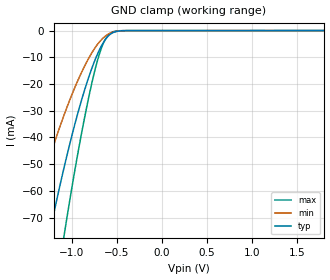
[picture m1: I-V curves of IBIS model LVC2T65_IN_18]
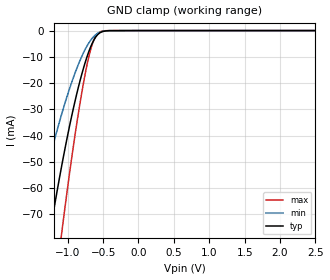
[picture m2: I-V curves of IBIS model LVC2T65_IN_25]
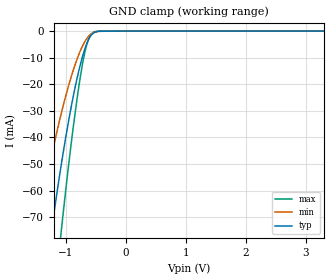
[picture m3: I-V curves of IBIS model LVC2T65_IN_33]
| TEXAS INSTRUMENTS INCORPORATED
| 2-BIT BIDIRECTIONAL VOLTAGE LEVEL TRANSLATOR FOR OPEN DRAIN APPLICATIONS
| Marketing part#   Voltage Range   Package-type   #pins/pkg drawing
| TXS0102DCU   1.65V - 5.5V   TSSOP   8 / DCU
| TXS0102DCT   1.65V - 5.5V   TSSOP   8 / DCT
| TXS0102DQE   1.65V - 5.5V   X2SON   8 / DQE
[IBIS Ver]   3.2
[File Name]   txs0102.ibs
[File Rev]   1.2
[Date]   May 11, 2015
[Source]   Model built from spectre simulations at:
   Texas Instruments Incorporated.
   Webench Design Center
   12500 TI Blvd
   Dallas, TX -75243
   For Support e-mail: elab_ibis@list.ti.com
[Notes]   Revision_History:
   Rev 1.2: Added DGE package component. 5/11/15
   Rev 1.1: Updated Vih/Vih for all buffers. 8/22/12
   Power Clamps and Pullups for IO_A and IO_B are non-monotonic
[Disclaimer] This model is designed as an aid for customers of Texas Instruments
 TI and its licensors and suppliers make no warranties, either expressed
 or implied, with respect to this  model, including the warranties of
 merchantability or fitness for a particular purpose.
 The model is provided solely on an "as is" basis. The entire risk as to
 its quality and performance is with the customer.
[Copyright] (C)Copyright 2015 Texas Instruments Incorporated.
   All rights reserved.
| Component TXS0102_DCU 8-PIN TSSOP
[Component]   TXS0102_DCU
[Manufacturer]   Texas Instruments, Inc.
[Package]
|   typ   min   max
R_pkg   1.400e-02   1.300e-02   1.500e-02
L_pkg   1.289e-09   1.025e-09   2.014e-09
C_pkg   1.360e-13   6.600e-14   2.940e-13
[Pin]   signal_name   model_name   R_pin   L_pin   C_pin
1   B2   LVC2T65_IO_B   1.400e-02   1.387e-09   1.760e-13
2   GND   GND   1.300e-02   1.026e-09   6.600e-14
3   VCCA   POWER   1.300e-02   1.032e-09   6.700e-14
4   A2   LVC2T65_IO_A   1.500e-02   2.014e-09   2.940e-13
5   A1   LVC2T65_IO_A   1.400e-02   1.412e-09   1.780e-13
6   OE   LVC2T65_IN   1.300e-02   1.030e-09   6.600e-14
7   VCCB   POWER   1.300e-02   1.025e-09   6.600e-14
8   B1   LVC2T65_IO_B   1.400e-02   1.386e-09   1.760e-13
| Component TXS0102_DCT 8-PIN TSSOP
[Component]   TXS0102_DCT
[Manufacturer]   Texas Instruments, Inc.
[Package]
|   typ   min   max
R_pkg   2.900e-02   2.800e-02   3.100e-02
L_pkg   1.796e-09   1.666e-09   1.924e-09
C_pkg   1.090e-13   8.300e-14   1.360e-13
[Pin]   signal_name   model_name   R_pin   L_pin   C_pin
1   B2   LVC2T65_IO_B   3.100e-02   1.894e-09   1.340e-13
2   GND   GND   2.800e-02   1.697e-09   8.600e-14
3   VCCA   POWER   3.000e-02   1.722e-09   8.600e-14
4   A2   LVC2T65_IO_A   3.000e-02   1.861e-09   1.300e-13
5   A1   LVC2T65_IO_A   2.800e-02   1.924e-09   1.360e-13
6   OE   LVC2T65_IN   2.900e-02   1.736e-09   8.600e-14
7   VCCB   POWER   2.800e-02   1.666e-09   8.300e-14
8   B1   LVC2T65_IO_B   3.000e-02   1.871e-09   1.320e-13
| Component TXS0102_DQE 8-PIN X2SON
[Component]   TXS0102_DQE
[Manufacturer]   Texas Instruments, Inc.
[Package]
|   typ   min   max
R_pkg   0.0401   0.0391   0.0417
L_pkg   0.3040n   0.2971n   0.3158n
C_pkg   0.0474p   0.0450p   0.0526p
[Pin]   signal_name   model_name   R_pin   L_pin   C_pin
1   VCCA   POWER   0.04056   0.31110n   0.04603p
2   A1   LVC2T65_IO_A   0.03969   0.30316n   0.04651p
3   A2   LVC2T65_IO_A   0.03995   0.30556n   0.05161p
4   GND   GND   0.03907   0.29711n   0.04499p
5   OE   LVC2T65_IN   0.03987   0.29814n   0.04522p
6   B2   LVC2T65_IO_B   0.03990   0.29821n   0.04651p
7   B1   LVC2T65_IO_B   0.04172   0.31579n   0.05261p
8   VCCB   POWER   0.04034   0.30276n   0.04549p
| Model LVC2T65_IN
[Model Selector]   LVC2T65_IN
LVC2T65_IN_18   1.8 volt Vcc
LVC2T65_IN_25   2.5 volt Vcc
LVC2T65_IN_33   3.3 volt Vcc
LVC2T65_IN_50   5 volt Vcc
| Model LVC2T65_IO_A
[Model Selector]   LVC2T65_IO_A
LVC2T65_IO_A_18   1.8 volt Vcc
LVC2T65_IO_A_25   2.5 volt Vcc
LVC2T65_IO_A_33   3.3 volt Vcc
LVC2T65_IO_A_50   5 volt Vcc
| Model LVC2T65_IO_B
[Model Selector]   LVC2T65_IO_B
LVC2T65_IO_B_18   1.8 volt Vcc
LVC2T65_IO_B_25   2.5 volt Vcc
LVC2T65_IO_B_33   3.3 volt Vcc
LVC2T65_IO_B_50   5 volt Vcc
| Models and submodels in the file (12): LVC2T65_IN_18 (Input), LVC2T65_IN_25 (Input), LVC2T65_IN_33 (Input), LVC2T65_IN_50 (Input), LVC2T65_IO_A_18 (I/O), LVC2T65_IO_A_25 (I/O), LVC2T65_IO_A_33 (I/O), LVC2T65_IO_A_50 (I/O), LVC2T65_IO_B_18 (I/O), LVC2T65_IO_B_25 (I/O), LVC2T65_IO_B_33 (I/O), LVC2T65_IO_B_50 (I/O)
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[Model]   LVC2T65_IN_18
Model_type  Input
Vinl=0.5775
Vinh=1.2675
| variable   typ   min   max
C_comp   3.03pF   2.64pF   3.31pF
[Temperature Range]   40   100   -40
| Ambient temperature   25   85   -40
[Voltage range]   1.8   1.65   1.95
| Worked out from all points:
|   GND clamp passes 1 mA (typ) near -0.55 V on its own axis
[GND Clamp]
| LVC2T65_IN_18
|   Voltage   I(typ)   I(min)   I(max)
-1.8V     -178.8mA   -117.9mA   -253.6mA
-1.5V     -120.5mA   -77.46mA   -175.4mA
-1.45V    -111.4mA   -71.26mA   -162.8mA
-1.24V    -75.33mA   -47.22mA   -111.9mA
-1.08V    -50.85mA   -31.35mA   -76.13mA
-1.06V    -48.01mA   -29.53mA   -71.89mA
-920mV    -29.69mA   -17.93mA   -44.11mA
-780mV    -14.62mA   -8.629mA   -20.46mA
-685mV    -6.852mA   -4.046mA   -8.189mA
-595mV    -2.137mA   -1.387mA   -1.816mA
-435mV    -62.85uA   -64.47uA   -17.43uA
1.8V      101.5pA    525.2pA    12.95pA
[Model]   LVC2T65_IN_25
Model_type  Input
Vinl=0.805
Vinh=1.755
| variable   typ   min   max
C_comp   2.96pF   2.56pF   3.28pF
[Temperature Range]   40   100   -40
| Ambient temperature   25   85   -40
[Voltage range]   2.5   2.3   2.7
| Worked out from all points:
|   GND clamp passes 1 mA (typ) near -0.55 V on its own axis
[GND Clamp]
| LVC2T65_IN_25
|   Voltage   I(typ)   I(min)   I(max)
-2.5V     -329.7mA   -228mA     -446.3mA
-1.49V    -118.7mA   -76.2mA    -172.8mA
-1.245V   -76.14mA   -47.75mA   -113.1mA
-1.095V   -53.01mA   -32.74mA   -79.35mA
-1.075V   -50.13mA   -30.89mA   -75.07mA
-905mV    -27.91mA   -16.82mA   -41.36mA
-825mV    -19.06mA   -11.33mA   -27.53mA
-740mV    -11.06mA   -6.498mA   -14.74mA
-650mV    -4.661mA   -2.806mA   -5.017mA
-600mV    -2.317mA   -1.49mA    -2.019mA
-545mV    -849.8uA   -621.1uA   -540.2uA
2.5V      135.7pA    628.3pA    18.04pA
[Model]   LVC2T65_IN_33
Model_type  Input
Vinl=1.05
Vinh=2.34
| variable   typ   min   max
C_comp   2.90pF   2.48pF   3.28pF
[Temperature Range]   40   100   -40
| Ambient temperature   25   85   -40
[Voltage range]   3.3   3   3.6
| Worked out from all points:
|   GND clamp passes 1 mA (typ) near -0.55 V on its own axis
[GND Clamp]
| LVC2T65_IN_33
|   Voltage   I(typ)   I(min)   I(max)
-3.3V     -515.1mA   -369.9mA   -673.8mA
-1.49V    -118.7mA   -76.2mA    -172.8mA
-1.245V   -76.14mA   -47.75mA   -113.1mA
-1.22V    -72.11mA   -45.11mA   -107.3mA
-1.085V   -51.57mA   -31.81mA   -77.2mA
-1.065V   -48.71mA   -29.98mA   -72.95mA
-895mV    -26.74mA   -16.09mA   -39.55mA
-740mV    -11.06mA   -6.498mA   -14.74mA
-640mV    -4.115mA   -2.5mA     -4.272mA
-580mV    -1.656mA   -1.109mA   -1.298mA
-525mV    -556.5uA   -430.2uA   -310.8uA
3.3V      182.2pA    758.6pA    23.96pA
